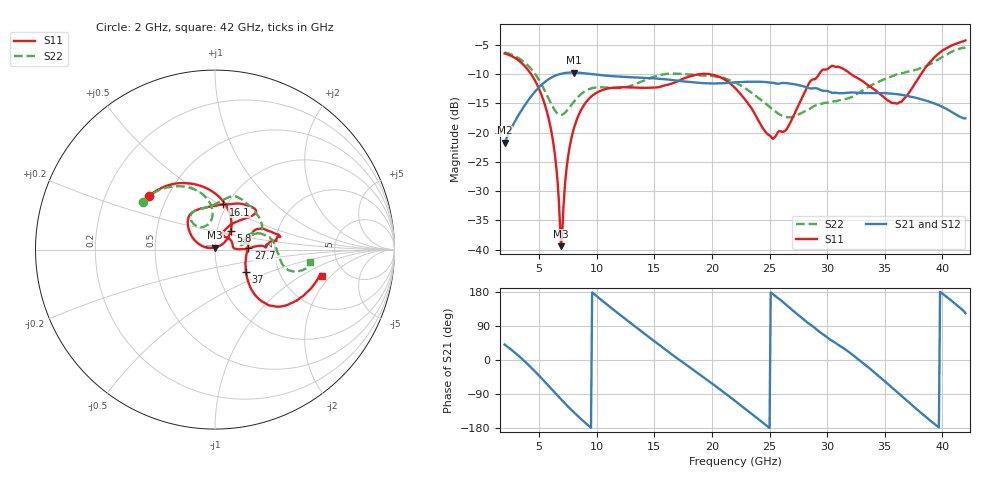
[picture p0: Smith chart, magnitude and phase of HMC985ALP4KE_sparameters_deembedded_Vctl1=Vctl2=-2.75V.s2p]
!s2p File: Measurements: S11, S21, S12, S22
# GHz S dB R 50.0
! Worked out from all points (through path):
!   401 points, 2 GHz to 42 GHz, reference 50 ohm
!   highest |S21| = -9.75 dB at 8 GHz (marker M1); lowest = -21.8 dB at 2 GHz (marker M2)
!   lowest |S11| = -39.4 dB at 6.9 GHz (marker M3), VSWR 1.02, Z = 50 + j1.07 ohm
!   |S11| at or under -10 dB: 4.289 GHz to 19.12 GHz (14.83 GHz wide, 127 % of centre); 19.71 GHz to 29.32 GHz (9.605 GHz wide, 39.2 % of centre); 32.05 GHz to 38.15 GHz (6.11 GHz wide, 17.4 % of centre)
!   |S22| runs from -17.4 to -5.5 dB; largest |S21 - S12| = 0.00035
!   S11 on the Smith chart (normalised r, x): 2 GHz: 0.40, +0.31; 5.8 GHz: 1.16, +0.24; 16.1 GHz: 0.96, +0.52; 27.7 GHz: 1.46, +0.02; 37 GHz: 1.36, -0.35; 42 GHz: 3.35, -1.57
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2  -6.49 140.6  -21.76 40.9  -21.76 40.9  -6.33 146.4
4.3  -10.03 90.4  -13.84 -19.7  -13.84 -19.7  -9.13 108.0
5.8  -17.42 49.6  -10.93 -67.6  -10.93 -67.7  -14.10 93.8
6.3  -22.77 38.4  -10.38 -84.2  -10.38 -84.2  -16.00 99.2
6.9  -39.41 89.9  -9.97 -103.7  -9.97 -103.8  -17.00 113.8
7.1  -33.09 157.4  -9.88 -110.1  -9.89 -110.1  -16.84 118.7
7.5  -24.27 165.8  -9.78 -122.6  -9.79 -122.6  -16.04 125.9
8  -19.40 158.6  -9.75 -137.6  -9.76 -137.6  -14.77 129.7
8.7  -15.94 148.0  -9.83 -157.5  -9.84 -157.5  -13.34 128.7
12.3  -12.26 118.9  -10.49 112.6  -10.50 112.6  -12.33 97.5
15.4  -12.24 88.8  -10.82 40.2  -10.83 40.2  -10.22 73.5
16.1  -11.86 79.9  -10.93 24.1  -10.94 24.1  -9.98 70.2
18.6  -10.14 50.6  -11.47 -31.0  -11.47 -31.0  -10.16 51.5
22  -12.38 46.0  -11.44 -107.8  -11.45 -107.8  -11.44 21.7
25.2  -20.94 56.6  -11.49 175.8  -11.49 175.8  -15.93 17.7
27.7  -14.59 2.4  -11.98 113.3  -11.98 113.3  -16.74 9.8
28.7  -10.97 2.3  -12.46 90.4  -12.47 90.4  -15.66 11.0
31.1  -8.85 13.5  -13.29 37.5  -13.30 37.5  -14.49 21.6
35.4  -14.67 6.4  -13.32 -66.7  -13.32 -66.7  -10.58 15.1
37  -13.50 -35.6  -13.77 -109.3  -13.77 -109.2  -9.62 6.6
39.6  -6.67 -43.2  -15.26 -175.5  -15.27 -175.5  -7.58 -15.3
42  -4.28 -13.9  -17.58 123.4  -17.58 123.4  -5.48 -7.5
